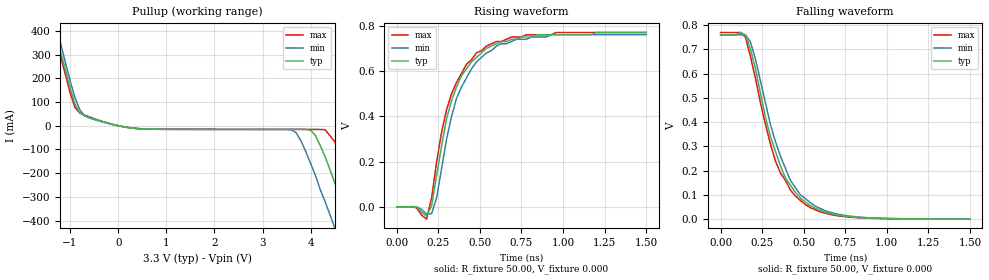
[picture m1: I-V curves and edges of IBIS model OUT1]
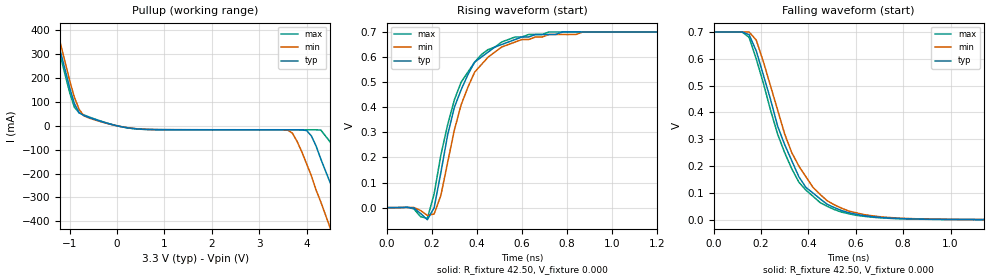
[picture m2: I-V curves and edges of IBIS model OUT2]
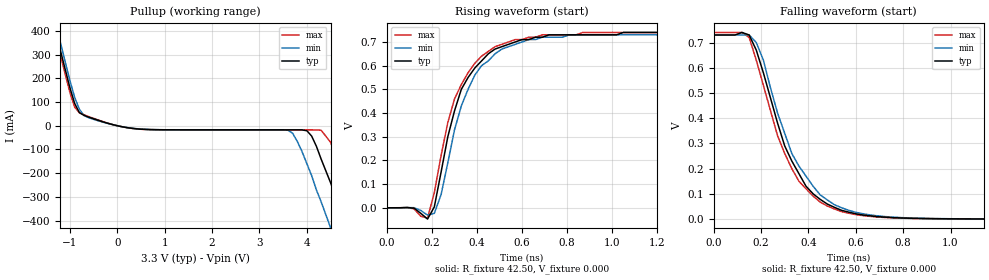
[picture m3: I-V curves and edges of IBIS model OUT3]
| Integrated Devices Technolgy, Inc
[Ibis Ver]   3.2
[File Name]   9zx21901b.ibs
[File Rev]   1.1
[Date]   11/10/2009
[Source]   Integrated Devices Technolgy, Inc.
|[Notes]   Rev 1.0 created by yfeng
[Notes]   Rev 1.1 added Vref, Rref, Vmeas
[Disclaimer] Integrated Device Technology, Inc. ("IDT") hereby grants the
   user of this IBIS model a non-exclusive, nontransferable
   license to use this IBIS model under the following terms. The
   user is granted this license only to use the IBIS model and is
   not granted rights to sell, copy (except as needed to run the
   IBIS model), rent, lease or sub-license the IBIS model in
   whole or in part, or in modified form to anyone. The User may
   modify the IBIS model to suit its specific applications, but
   rights to derivative works and such modifications shall belong
   to IDT. This IBIS model is provided on an AS IS" basis and IDT
   makes absolutely no warranty with respect to the information
   contained herein. IDT DISCLAIMS AND CUSTOMER WAIVES ALL
   WARRANTIES, EXPRESS AND IMPLIED, INCLUDING WARRANTIES OF
   MERCHANTABILITY AND FITNESS FOR A PARTICULAR PURPOSE. THE
   ENTIRE RISK AS TO QUALITY AND PERFORMANCE IS WITH THE USER
   ACCORDINGLY, IN NO EVENT SHALL IDT BE LIABLE FOR ANY DIRECT OR
   INDIRECT DAMAGES, WHETHER IN CONTRACT OR TORT, INCLUDING ANY
   LOST PROFITS OR OTHER INCIDENTAL, CONSEQUENTIAL, EXEMPLARY, OR
   PUNITIVE DAMAGES ARISING OUT OF THE USE OR APPLICATION OF THE
   IBIS model. Further, IDT reserves the right to make changes
   without notice to any product herein to improve reliability,
   function, or design. IDT does not convey any license under
   patent rights or any other intellectual property rights,
   including those of third parties. IDT is not obligated to
   provide maintenance or support for the licensed IBIS model.
[Disclaimer]   (C) Copyright Integrated Device Technology, Inc. 2007 All
   rights reserved
|   COMPONENT: ICS9ZX21901b
[Component]   ICS9ZX21901b
[Manufacturer]   Integrated Device Technology, Inc.
[Package]
| variable   typ   min   max
R_pkg   81.10m   62.20m   100.00m
L_pkg   6.70nH   4.90nH   8.50nH
C_pkg   0.53pF   0.21pF   0.85pF
[Pin]   signal_name   model_name   R_pin   L_pin   C_pin
1   VDDA   POWER
2   GNDA   GND
3   IREF   OUT
4   100M_133M#   IN
5   HIBW_BYPM_LOBW#   IN
6   CK_POWERGD/PD#   IN
7   GND   GND
8   VDD   POWER
9   DIF_IN   IN
10   DIF_IN#   IN
11   SMB_A0_tri   IN
12   SMBDAT   IO_D
13   SMBCLK   IN_D
14   SMB_A1_tri   IN
15   DFB_IN   IN
16   DFB_IN#   IN
17   DFB_OUT#   OUT
18   DFB_OUT   OUT
19   DIF_0   OUT
20   DIF_0#   OUT
21   VDD   POWER
22   DIF_1   OUT
23   DIF_1#   OUT
24   DIF_2   OUT
25   DIF_2#   OUT
26   GND   GND
27   DIF_3   OUT
28   DIF_3#   OUT
29   DIF_4   OUT
30   DIF_4#   OUT
31   VDD   POWER
32   DIF_5   OUT
33   DIF_5#   OUT
34   OE5#   IN
35   DIF_6   OUT
36   DIF_6#   OUT
37   OE6#   IN
38   DIF_7   OUT
39   DIF_7#   OUT
40   OE7#   IN
41   DIF_8   OUT
42   DIF_8#   OUT
43   OE8#   IN
44   GND   GND
45   VDD   POWER
46   DIF_9   OUT
47   DIF_9#   OUT
48   OE9#   IN
49   DIF_10   OUT
50   DIF_10#   OUT
51   OE10#   IN
52   DIF_11   OUT
53   DIF_11#   OUT
54   OE_11#   IN
55   DIF_12   OUT
56   DIF_12#   OUT
57   OE12#   IN
58   VDD   POWER
59   DIF_13   OUT
60   DIF_13#   OUT
61   DIF_14   OUT
62   DIF_14#   OUT
63   GND   GND
64   DIF_15   OUT
65   DIF_15#   OUT
66   DIF_16   OUT
67   DIF_16#   OUT
68   VDD   POWER
69   DIF_17   OUT
70   DIF_17#   OUT
71   DIF_18   OUT
72   DIF_18#   OUT
[Diff Pin]   inv_pin   vdiff   tdelay_typ
9   10   NA   NA
15   16   NA   NA
18   17   NA   NA
19   20   NA   NA
22   23   NA   NA
24   25   NA   NA
27   28   NA   NA
29   30   NA   NA
32   33   NA   NA
35   36   NA   NA
38   39   NA   NA
41   42   NA   NA
46   47   NA   NA
49   50   NA   NA
52   53   NA   NA
55   56   NA   NA
59   60   NA   NA
61   62   NA   NA
64   65   NA   NA
66   67   NA   NA
69   70   NA   NA
71   72   NA   NA
[Model Selector] OUT
OUT1   100ohm differential output trace. 475ohm on IREF pin.
OUT2   85ohm differential output trace. 432ohm on IREF pin.
OUT3   85ohm differential output trace. 412ohm on IREF pin.
| Models and submodels in the file (6): OUT1 (Open_source), OUT2 (Open_source), OUT3 (Open_source), IN (Input), IO_D (I/O_open_drain), IN_D (Input)
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|   Model OUT1
[Model]   OUT1
Model_type   Open_source
Polarity   Non-Inverting
Vmeas =  0.350V
Cref =   2.00pF
Rref =  50.000
Vref =   0.350V
Enable   Active-High
C_comp   3.40pF   2.85pF   3.95pF
[Temperature Range]   27.00   70.00   0.000
[Voltage Range]   3.30V   3.00V   3.60V
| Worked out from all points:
|   slope of the pullup table from 0 to 0.495 V, typ, clamps not added: 37.6 ohm
|   rising waveform, R_fixture 50.00, V_fixture 0.000: 20-80 % time 183ps typ, 183ps min, 178ps max; typ from 0 V to 0.77 V
|   falling waveform, R_fixture 50.00, V_fixture 0.000: 20-80 % time 194ps typ, 201ps min, 196ps max; typ from 0.76 V to 0 V
[Pullup]
| voltage   I(typ)   I(min)   I(max)
-3.3V     2.06A      2.09A      2.05A
-1.5V     550mA      590mA      530mA
-900mV    93.18mA    120mA      77.76mA
-500mV    28.45mA    26.28mA    30.19mA
3.6V      -15.31mA   -16.83mA   -15.36mA
4V        -18.89mA   -160mA     -15.37mA
4.3V      -130mA     -320mA     -16.85mA
4.5V      -240mA     -430mA     -67.51mA
4.7V      -350mA     -540mA     -170mA
4.9V      -460mA     -650mA     -280mA
5.1V      -580mA     -760mA     -400mA
6.6V      -1.44A     -1.6A      -1.27A
[Ramp]
| variable   typ   min   max
dV/dt_r   0.46/0.18n   0.46/0.18n   0.46/0.17n
dV/dt_f   0.46/0.20n   0.46/0.20n   0.46/0.19n
R_load = 50.00
[Rising Waveform]
R_fixture = 50.00
V_fixture = 0.000
V_fixture_min = 0.000
V_fixture_max = 0.000
| time   V(typ)   V(min)   V(max)
0s        52.45uV    49.42uV    57.25uV
120ps     -1.48mV    500uV      -4.67mV
180ps     -39.8mV    -32.47mV   -53.51mV
210ps     5.66mV     -29.54mV   41.27mV
240ps     140mV      40.56mV    200mV
300ps     390mV      300mV      430mV
360ps     530mV      480mV      550mV
480ps     660mV      640mV      680mV
720ps     740mV      740mV      750mV
1.5ns     770mV      760mV      770mV
[Falling Waveform]
R_fixture = 50.00
V_fixture = 0.000
V_fixture_min = 0.000
V_fixture_max = 0.000
| time   V(typ)   V(min)   V(max)
0s        760mV      760mV      770mV
120ps     770mV      760mV      770mV
150ps     760mV      760mV      750mV
180ps     700mV      730mV      670mV
270ps     420mV      480mV      390mV
330ps     280mV      320mV      240mV
420ps     140mV      160mV      120mV
510ps     70.41mV    84.41mV    60.12mV
780ps     9.22mV     11.83mV    7.74mV
1.5ns     66.75uV    97.12uV    35.69uV
|   Model OUT2
[Model]   OUT2
Model_type   Open_source
Polarity   Non-Inverting
Enable   Active-High
Vmeas =  0.350V
Cref =   2.00pF
Rref =  50.000
Vref =   0.350V
C_comp   3.40pF   2.85pF   3.95pF
[Temperature Range]   27.00   70.00   0.000
[Voltage Range]   3.30V   3.00V   3.60V
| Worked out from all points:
|   slope of the pullup table from 0 to 0.495 V, typ, clamps not added: 35.5 ohm
|   rising waveform, R_fixture 42.50, V_fixture 0.000: 20-80 % time 138ps typ, 149ps min, 149ps max; typ from 0 V to 0.7 V
|   falling waveform, R_fixture 42.50, V_fixture 0.000: 20-80 % time 172ps typ, 185ps min, 167ps max; typ from 0.7 V to 0 V
[Pullup]
| voltage   I(typ)   I(min)   I(max)
-3.3V     2.06A      2.09A      2.05A
-1.5V     550mA      590mA      530mA
-900mV    93.48mA    120mA      78.18mA
-500mV    28.92mA    26.72mA    30.68mA
500mV     -13.95mA   -13.46mA   -14.27mA
3.6V      -16.51mA   -18.02mA   -16.56mA
4V        -20.09mA   -160mA     -16.57mA
4.3V      -140mA     -320mA     -18.05mA
4.5V      -240mA     -430mA     -68.71mA
4.9V      -470mA     -650mA     -280mA
5.1V      -580mA     -760mA     -400mA
6.6V      -1.44A     -1.6A      -1.27A
[Ramp]
| variable   typ   min   max
dV/dt_r   0.49/0.18n   0.49/0.19n   0.50/0.18n
dV/dt_f   0.49/0.19n   0.49/0.20n   0.50/0.19n
R_load = 50.00
[Rising Waveform]
R_fixture = 42.50
V_fixture = 0.000
V_fixture_min = 0.000
V_fixture_max = 0.000
| time   V(typ)   V(min)   V(max)
0s        51.6uV     48.65uV    56.35uV
120ps     -1.67mV    460uV      -5.05mV
180ps     -48.04mV   -31.16mV   -42.6mV
210ps     -550uV     -25.45mV   54.69mV
270ps     290mV      180mV      330mV
330ps     470mV      410mV      500mV
390ps     580mV      540mV      580mV
510ps     650mV      640mV      660mV
870ps     700mV      700mV      700mV
1.5ns     700mV      700mV      700mV
[Falling Waveform]
R_fixture = 42.50
V_fixture = 0.000
V_fixture_min = 0.000
V_fixture_max = 0.000
| time   V(typ)   V(min)   V(max)
0s        700mV      700mV      700mV
120ps     700mV      700mV      700mV
150ps     690mV      700mV      680mV
180ps     630mV      670mV      600mV
270ps     350mV      410mV      320mV
330ps     220mV      250mV      190mV
390ps     120mV      160mV      110mV
450ps     77.34mV    94.08mV    63.61mV
720ps     7.36mV     9.45mV     6.14mV
1.5ns     41.6uV     45.49uV    -5.31uV
|   Model OUT3
[Model]   OUT3
Model_type   Open_source
Polarity   Non-Inverting
Enable   Active-High
Vmeas =  0.350V
Cref =   2.00pF
Rref =  50.000
Vref =   0.350V
C_comp   3.40pF   2.85pF   3.95pF
[Temperature Range]   27.00   70.00   0.000
[Voltage Range]   3.30V   3.00V   3.60V
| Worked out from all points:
|   slope of the pullup table from 0 to 0.495 V, typ, clamps not added: 34.2 ohm
|   rising waveform, R_fixture 42.50, V_fixture 0.000: 20-80 % time 152ps typ, 148ps min, 150ps max; typ from 0 V to 0.74 V
|   falling waveform, R_fixture 42.50, V_fixture 0.000: 20-80 % time 172ps typ, 185ps min, 171ps max; typ from 0.73 V to 0 V
[Pullup]
| voltage   I(typ)   I(min)   I(max)
-3.3V     2.06A      2.09A      2.05A
-1.5V     550mA      590mA      530mA
-900mV    93.67mA    120mA      78.44mA
-500mV    29.22mA    26.99mA    31mA
500mV     -14.45mA   -13.92mA   -14.8mA
3.6V      -17.3mA    -18.82mA   -17.36mA
4V        -20.89mA   -160mA     -17.37mA
4.3V      -140mA     -320mA     -18.85mA
4.5V      -240mA     -430mA     -69.51mA
4.9V      -470mA     -650mA     -280mA
5.1V      -580mA     -760mA     -400mA
6.6V      -1.44A     -1.61A     -1.27A
[Ramp]
| variable   typ   min   max
dV/dt_r   0.52/0.19n   0.52/0.19n   0.52/0.18n
dV/dt_f   0.52/0.20n   0.52/0.20n   0.52/0.19n
R_load = 50.00
[Rising Waveform]
R_fixture = 42.50
V_fixture = 0.000
V_fixture_min = 0.000
V_fixture_max = 0.000
| time   V(typ)   V(min)   V(max)
0s        51.6uV     48.65uV    56.35uV
120ps     -1.67mV    460uV      -4.69mV
180ps     -47.48mV   -30.79mV   -43.47mV
210ps     3.73mV     -23.28mV   63.75mV
270ps     300mV      190mV      360mV
330ps     500mV      430mV      520mV
390ps     590mV      560mV      610mV
480ps     670mV      650mV      680mV
810ps     730mV      730mV      730mV
1.5ns     740mV      730mV      740mV
[Falling Waveform]
R_fixture = 42.50
V_fixture = 0.000
V_fixture_min = 0.000
V_fixture_max = 0.000
| time   V(typ)   V(min)   V(max)
0s        730mV      730mV      740mV
120ps     740mV      730mV      740mV
150ps     730mV      730mV      720mV
180ps     670mV      700mV      630mV
270ps     380mV      420mV      330mV
330ps     230mV      260mV      200mV
390ps     130mV      170mV      120mV
480ps     59.35mV    75.72mV    51.54mV
750ps     6mV        7.86mV     4.91mV
1.5ns     58.66uV    38.86uV    990nV
